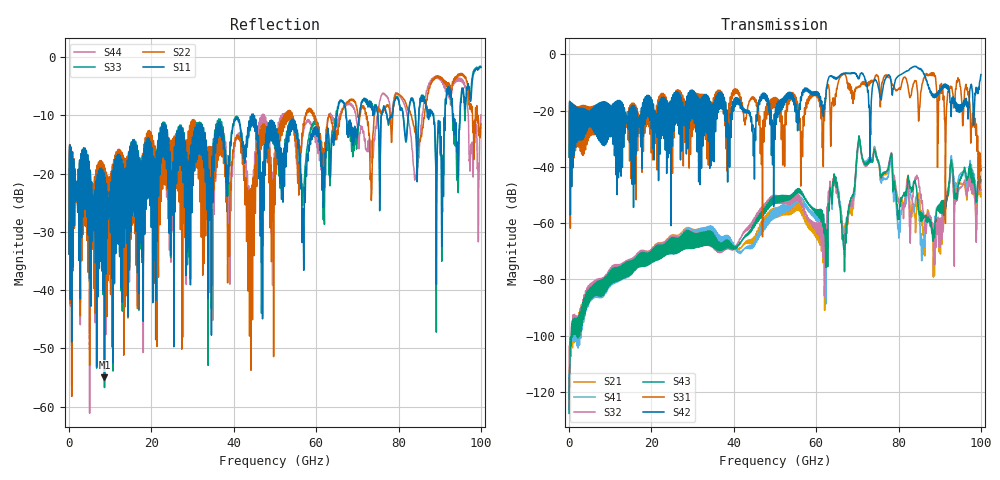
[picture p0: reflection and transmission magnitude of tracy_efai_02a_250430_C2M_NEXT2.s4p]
!! PART DESCRIPTION: TE 224G+ VSR Channel- Chip to module, IO connector to CPC(Co-packaged connector) through over the board cable
!! CHANNEL DESCRIPTION: Module trace -> Mated IO 224G+ Connector -> Internal Cable Termination -> 30AWG 300mm Cable -> Cable
!!  termination + CPC connector(No footprint or package included)
!! MODEL REVISION:  Rev 3, Created on April 29, 2025
!! MODEL STATUS: Development
!! MODEL GEOMETRY: NEXT2
!! MODEL FREQUENCY RANGE: 0 GHz to 100 GHz in 10.00 MHz frequency steps
!! PORT DEFINITIONS:
!! Port  1  ----->  Module Side  -->  Module Side  <-----  Port  2
!! Port  3  ----->  Module Side  -->  Module Side  <-----  Port  4
# HZ S MA R 45.000000
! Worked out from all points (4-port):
!   10000 points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, 10 MHz to 100 GHz, reference 45 ohm
!   strongest paths, dB at 10 MHz, 25.01 GHz, 50.01 GHz, 75.01 GHz, 100 GHz:
!     S42: -36.5, -18.1, -28.3, -11.1, -7.2
!     S31: -36.5, -17.8, -16.0, -7.7, -40.6
!     S43: -127.6, -70.8, -50.9, -37.7, -44.5
!     S32: -126.4, -70.2, -50.4, -38.4, -48.0
!     S41: -122.0, -70.2, -55.5, -37.7, -45.0
!     S21: -123.9, -69.6, -55.0, -38.2, -49.2
!   lowest |S11| = -54.9 dB at 8.6 GHz (marker M1), VSWR 1.00, Z = 44.9 + j0.15 ohm
!   |S11| at or under -10 dB: start of sweep to 44.32 GHz; 44.72 GHz to 64.9 GHz (20.18 GHz wide, 36.8 % of centre); 67.23 GHz to 70.41 GHz (3.185 GHz wide, 4.63 % of centre)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
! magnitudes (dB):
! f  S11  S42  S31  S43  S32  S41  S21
! 10 MHz  -33.8  -36.5  -36.5  -127.6  -126.4  -122.0  -123.9
! 8.6 GHz  -54.9  -28.3  -27.5  -82.9  -82.1  -83.6  -82.5
! 64.52 GHz  -14.1  -8.1  -18.1  -45.3  -46.3  -45.0  -45.9
! 66.8 GHz  -7.9  -6.7  -7.1  -71.2  -66.3  -65.4  -61.8
! 70.49 GHz  -9.9  -8.3  -11.3  -29.8  -29.8  -30.3  -30.3
! 88.17 GHz  -9.4  -13.8  -7.5  -62.7  -60.3  -61.6  -64.0
! 100 GHz  -1.8  -7.2  -40.6  -44.5  -48.0  -45.0  -49.2
